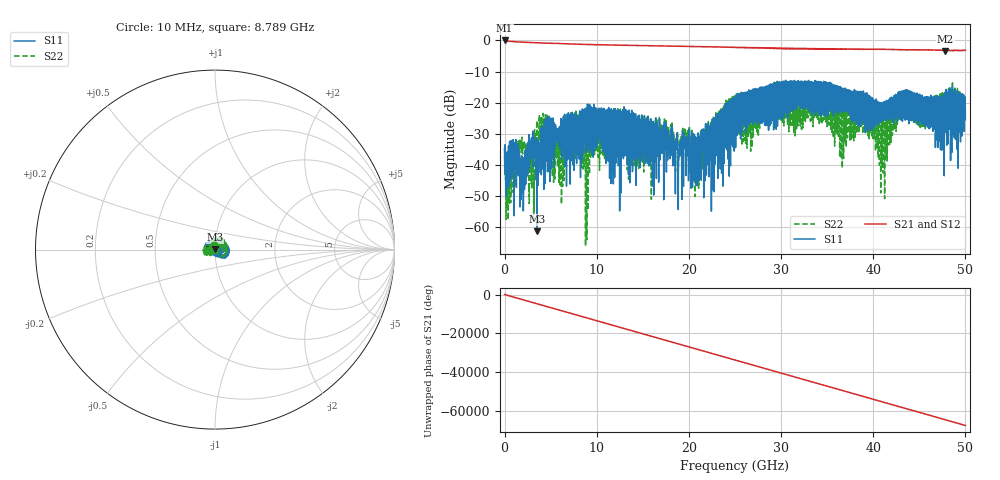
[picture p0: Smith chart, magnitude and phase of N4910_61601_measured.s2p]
!Keysight Technologies,N5245A,MY49151038,A.09.90.19
!Keysight N5245A: A.09.90.19
!Date: Wednesday, September 06, 2017 03:31:17
!Correction: S11(Full 4 Port(1,2,3,4))
!S21(Full 4 Port(1,2,3,4))
!S12(Full 4 Port(1,2,3,4))
!S22(Full 4 Port(1,2,3,4))
!S2P File: Measurements: S11, S21, S12, S22:
# Hz S  dB  R 50
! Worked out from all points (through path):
!   3201 points, 10 MHz to 50 GHz, reference 50 ohm
!   highest |S21| = 0.00 dB at 10 MHz (marker M1); lowest = -3.4 dB at 47.83 GHz (marker M2)
!   group delay of S21, straight-line fit = 3.76 ns
!   lowest |S11| = -61.3 dB at 3.509 GHz (marker M3), VSWR 1.00, Z = 50 + j0.0847 ohm
!   |S11| at or under -10 dB: start of sweep to end of sweep
!   |S22| runs from -66.0 to -12.8 dB; largest |S21 - S12| = 0.013
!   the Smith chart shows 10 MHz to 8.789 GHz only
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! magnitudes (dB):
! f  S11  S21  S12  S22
! 10 MHz  -34.8  0.0  0.1  -34.3
! 416.2 MHz  -35.3  -0.2  -0.2  -52.8
! 1.322 GHz  -35.2  -0.4  -0.4  -38.4
! 1.916 GHz  -46.9  -0.5  -0.5  -32.9
! 2.916 GHz  -31.5  -0.7  -0.6  -44.9
! 3.509 GHz  -61.3  -0.7  -0.7  -26.0
! 4.665 GHz  -42.1  -0.9  -0.9  -28.7
! 5.962 GHz  -29.7  -1.0  -1.0  -30.8
! 6.993 GHz  -37.7  -1.1  -1.1  -32.8
! 8.352 GHz  -28.2  -1.2  -1.2  -30.9
! 16.68 GHz  -29.6  -1.7  -1.8  -28.0
! 18.74 GHz  -29.6  -1.8  -1.9  -29.3
! 19.69 GHz  -43.4  -1.9  -1.9  -33.4
! 20.88 GHz  -34.3  -2.0  -2.0  -34.5
! 25 GHz  -18.2  -2.3  -2.2  -17.8
! 33.35 GHz  -20.6  -2.6  -2.6  -21.5
! 39.14 GHz  -29.6  -2.8  -2.8  -29.5
! 41.02 GHz  -20.4  -2.8  -2.9  -21.7
! 41.67 GHz  -24.0  -2.9  -2.9  -27.6
! 43.31 GHz  -24.8  -2.9  -2.9  -24.9
! 47.83 GHz  -27.2  -3.4  -3.4  -20.8
! 50 GHz  -25.4  -3.2  -3.1  -24.0
